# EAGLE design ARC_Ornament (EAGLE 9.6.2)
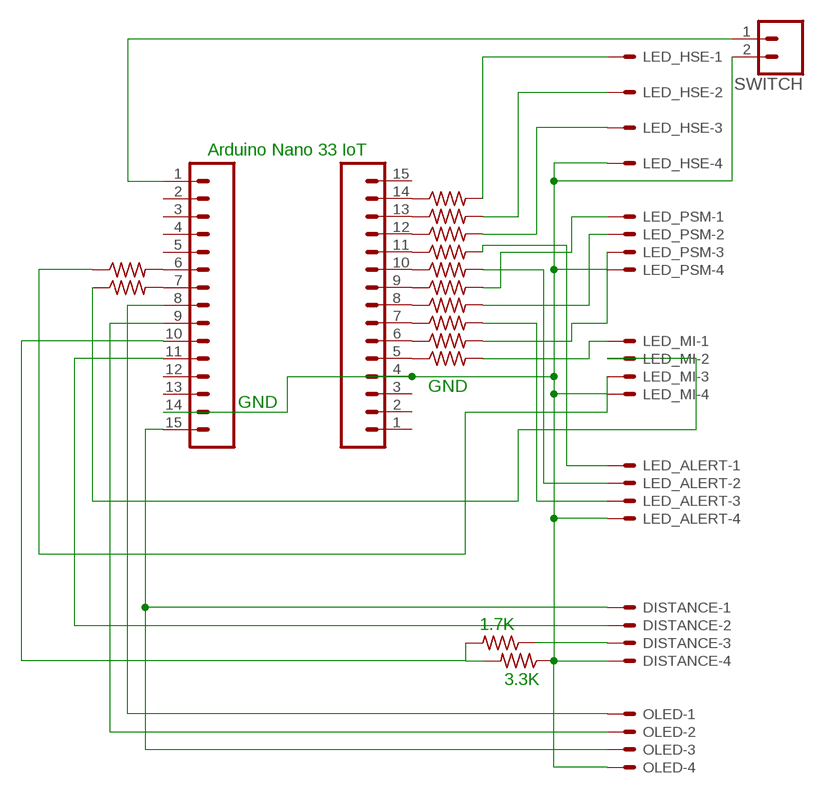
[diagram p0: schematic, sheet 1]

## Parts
1K7  R-US_0204/7  [0204/7]
3K3  R-US_0204/7  [0204/7]
DISTANCE  22-27-2041-04  [6410-04]
J1  CONN_15  [1X15]
J5  CONN_15  [1X15]
LED_ALERT  22-27-2041-04  [6410-04]
LED_HSE  22-27-2041-04  [6410-04]
LED_MI  22-27-2041-04  [6410-04]
LED_PSM  22-27-2041-04  [6410-04]
OLED  22-27-2041-04  [6410-04]
R1  R-US_0204/7  [0204/7]
R2  R-US_0204/7  [0204/7]
R3  R-US_0204/7  [0204/7]
R4  R-US_0204/7  [0204/7]
R5  R-US_0204/7  [0204/7]
R6  R-US_0204/7  [0204/7]
R7  R-US_0204/7  [0204/7]
R8  R-US_0204/7  [0204/7]
R9  R-US_0204/7  [0204/7]
R10  R-US_0204/7  [0204/7]
R11  R-US_0204/7  [0204/7]
R12  R-US_0204/7  [0204/7]
SWITCH  CONN_02  [1X02]

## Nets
GND: 3K3.1 DISTANCE.4 J1.4 J5.14 LED_ALERT.4 LED_HSE.4 LED_MI.4 LED_PSM.4 OLED.4 SWITCH.2
N$1: J1.5 R1.1
N$3: LED_HSE.1 R7.2
N$6: J1.6 R2.1
N$7: J1.8 R3.1
N$8: J1.9 R4.1
N$9: J1.12 R5.1
N$10: J1.13 R6.1
N$11: J1.14 R7.1
N$12: LED_PSM.2 R3.2
N$13: J5.6 R9.2
N$14: J5.7 R10.2
N$15: LED_PSM.3 R2.2
N$16: LED_MI.1 R1.2
N$17: LED_MI.2 R10.1
N$18: LED_PSM.1 R4.2
N$19: LED_MI.3 R9.1
N$20: J1.11 R8.1
N$21: J1.10 R11.1
N$22: J1.7 R12.1
N$23: LED_ALERT.3 R12.2
N$24: LED_ALERT.2 R11.2
N$25: LED_ALERT.1 R8.2
N$26: J5.9 OLED.2
N$27: DISTANCE.1 J5.15 OLED.3
N$28: J5.8 OLED.1
N$29: J5.1 SWITCH.1
N$30: DISTANCE.2 J5.11
N$31: 1K7.2 3K3.2 J5.10
N$32: 1K7.1 DISTANCE.3
N$33: LED_HSE.2 R6.2
N$34: LED_HSE.3 R5.2
Unconnected: J1.1 J1.2 J1.3 J1.15 J5.2 J5.3 J5.4 J5.5 J5.12 J5.13

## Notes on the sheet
- Arduino Nano 33 IoT
- GND
- GND
- 1.7K
- 3.3K

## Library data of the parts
1K7 3K3 R1-R12 = rcl:R-US_: RESISTOR, American symbol; SPICEPREFIX: R
DISTANCE LED_ALERT LED_HSE LED_MI LED_PSM OLED = sean-4pin-molexbr:22-?-04: CONNECTOR wire to board 2.54 mm (.1 inch) pitch header; MF: MOLEX; OC_FARNELL: unknown; OC_NEWARK: unknown
J1 J5 = SparkFun-Connectors:CONN_15: Multi connection point. Often used as Generic Header-pin footprint for 0.1 inch spaced/style header connections On any of the 0.1 inch spaced packages, you can populate with these: Break Away Headers - Straight (PRT-00116) Break Away Male Headers - Right Angle (PRT-00553) Female Headers (PRT-00115)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
SWITCH = SparkFun-Connectors:CONN_02: Multi connection point. Often used as Generic Header-pin footprint for 0.1 inch spaced/style header connections

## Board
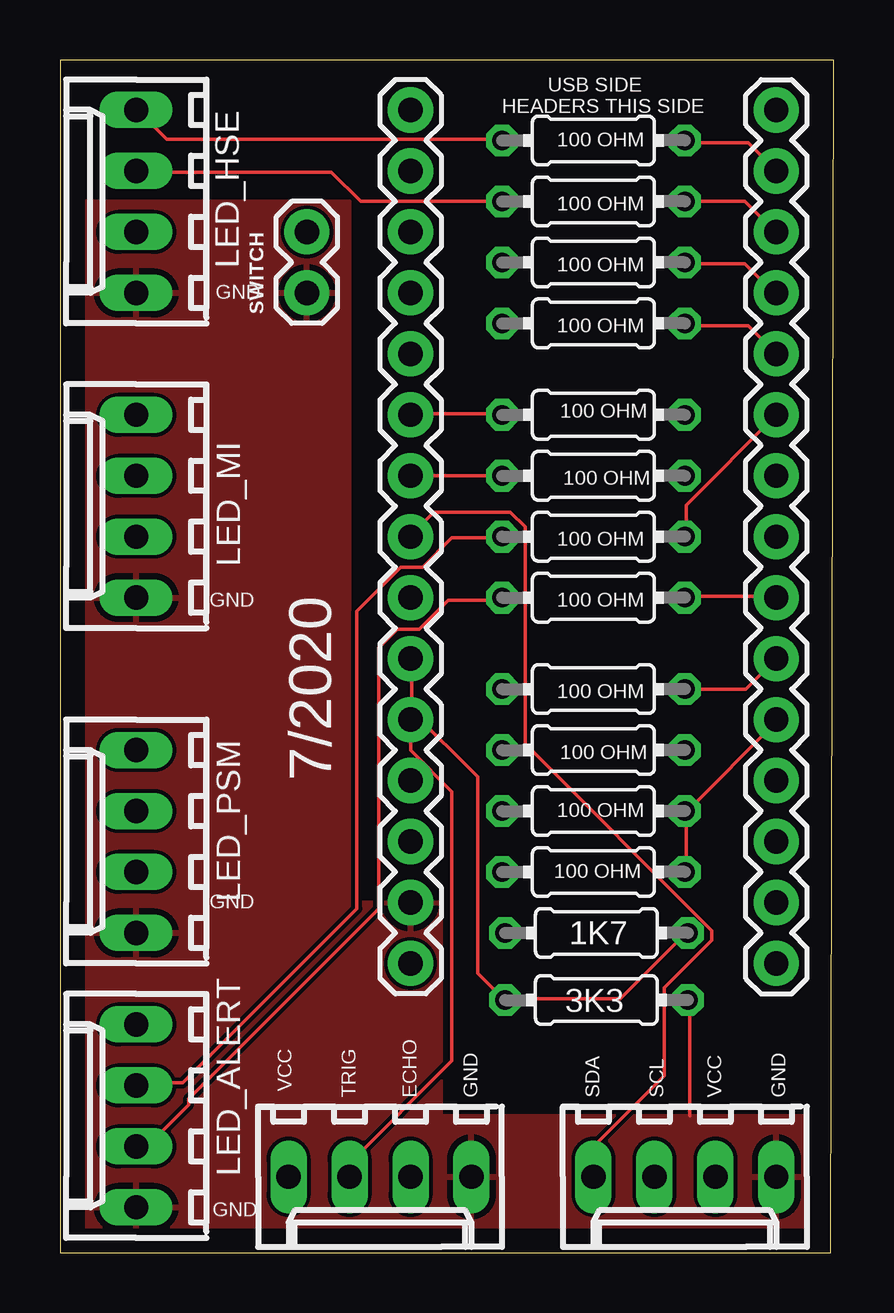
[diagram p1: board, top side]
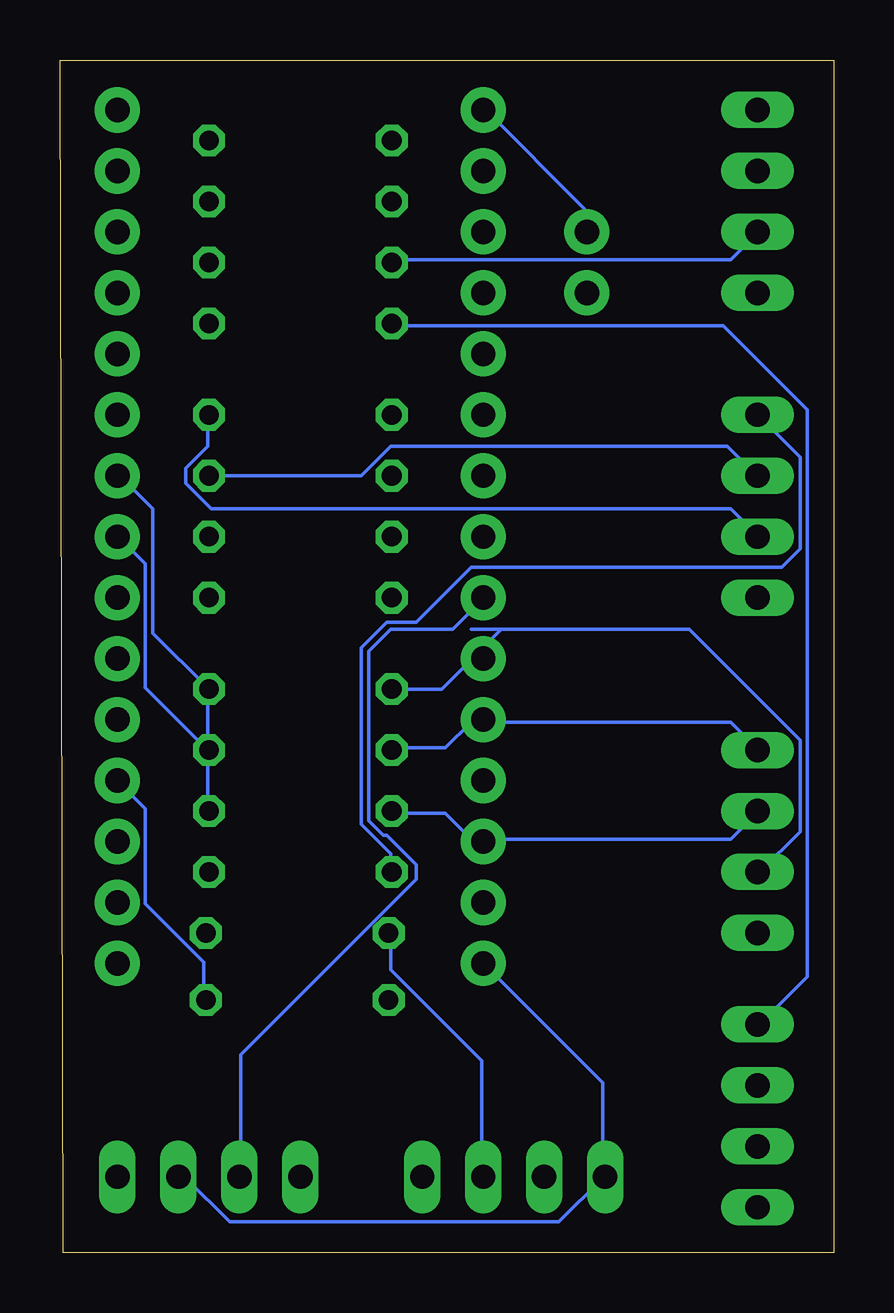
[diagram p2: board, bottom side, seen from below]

Size 32.24 x 49.71 mm. Coordinates in mm from the lower left corner, seen from the top.
Outline: 0,0 32.11,0 32.24,49.71 0,49.71 0,0
Copper layers (1*16): Top 0.035mm / dielectric 1.5mm / Bottom 0.035mm
Design rules "default": minimum track width 6mil, minimum drill 0.35mm, track to track 6mil, track to pad 6mil, pad to pad 6mil, via to via 6mil, smd to smd 6mil, copper to edge 40mil, drill to drill 6mil, minimum pad ring 10mil, minimum via ring 8mil, stop-mask expansion 4mil, vias tented up to drill 0mil, thermal gap 10mil

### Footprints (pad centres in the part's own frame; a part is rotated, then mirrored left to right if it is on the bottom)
0204/7 = drill 0.813 octagon: 1 -3.81,0; 2 3.81,0
6410-04 = drill 1.016 long: 1 3.81,0; 2 1.27,0; 3 -1.27,0; 4 -3.81,0
1X15 = drill 1.016 pad 1.88: 1 0,0; 2 2.54,0; 3 5.08,0; 4 7.62,0; 5 10.16,0; 6 12.7,0; 7 15.24,0; 8 17.78,0; 9 20.32,0; 10 22.86,0; 11 25.4,0; 12 27.94,0; 13 30.48,0; 14 33.02,0; 15 35.56,0
1X02 = drill 1.016 pad 1.88: 1 0,0; 2 2.54,0

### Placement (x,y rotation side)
1K7  22.35,13.34 0 top
3K3  22.35,10.54 180 top
DISTANCE  13.34,3.17 180 top
J1  29.84,12.06 90 top
J5  14.61,47.62 270 top
LED_ALERT  3.17,5.71 90 top
LED_HSE  3.17,43.81 90 top
LED_MI  3.17,31.12 90 top
LED_PSM  3.17,17.14 90 top
OLED  26.04,3.17 180 top
R1  22.23,15.88 180 top
R2  22.23,23.49 180 top
R3  22.23,18.41 180 top
R4  22.23,20.95 180 top
R5  22.23,41.27 180 top
R6  22.23,43.81 180 top
R7  22.23,46.35 180 top
R8  22.23,38.73 180 top
R9  22.23,34.93 180 top
R10  22.23,32.38 180 top
R11  22.23,29.84 180 top
R12  22.23,27.3 180 top
SWITCH  10.29,42.54 270 top

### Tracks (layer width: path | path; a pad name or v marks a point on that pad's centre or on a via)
GND
  Top 0.152: 26.24,5.71 26.24,10.44 3K3.1
  Bottom 0.152: J1.4 28.68,18.52 28.68,14.55 26.24,12.12 26.24,10.59 3K3.1
  pour Top: 0.63,0.63 31.12,0.63 31.12,5.71 15.88,5.71 15.88,14.6 12.07,14.6 12.07,43.81 0.63,43.81
N$1
  Top 0.152: R1.1 26.09,15.88 26.09,18.36 29.9,22.17 J1.5
N$3
  Top 0.152: R7.2 18.31,46.41 4.44,46.41 3.23,47.62 LED_HSE.1
N$6
  Top 0.152: J1.6 28.58,23.49 R2.1
N$7
  Bottom 0.152: R3.1 26.09,18.47 26.09,20.95 28.68,23.55 28.68,28.73 29.74,29.79 J1.8
N$8
  Bottom 0.152: R4.1 26.09,21.06 26.09,23.55 28.37,25.83 28.37,31.01 29.74,32.38 J1.9
N$9
  Top 0.152: R5.1 26.09,41.22 28.52,41.22 29.74,40.01 J1.12
N$10
  Top 0.152: R6.1 28.52,43.81 29.74,42.6 J1.13
N$11
  Top 0.152: J1.14 28.68,46.25 26.09,46.25 R7.1
N$12
  Bottom 0.152: R3.2 18.31,18.31 16.18,18.31 15.11,17.25 4.29,17.25 3.23,18.31 LED_PSM.2
N$13
  Top 0.152: R9.2 18.31,34.98 14.66,34.98 J5.6
N$14
  Top 0.152: J5.7 R10.2
N$15
  Bottom 0.152: R2.2 16.33,23.49 13.84,25.98 | 15.11,25.98 6.02,25.98 1.4,21.36 1.4,17.55 3.07,15.88 LED_PSM.3
N$16
  Bottom 0.152: LED_MI.1 1.4,33.15 1.4,29.34 2.16,28.57 15.11,28.57 17.4,26.29 18.62,26.29 19.69,25.22 19.69,17.86 18.47,16.64 18.47,15.88 R1.2
N$17
  Bottom 0.152: R10.1 19.69,32.38 18.47,33.6 4.44,33.6 3.23,32.38 LED_MI.2
N$18
  Bottom 0.152: R4.2 18.31,21.06 16.18,21.06 15.11,22.12 4.29,22.12 3.23,21.06 LED_PSM.1
N$19
  Bottom 0.152: R9.1 26.09,34.82 26.09,33.6 27,32.69 27,32.08 25.93,31.01 4.29,31.01 3.23,29.95 LED_MI.3
N$20
  Top 0.152: J1.11 28.68,38.63 26.09,38.63 R8.1
N$21
  Top 0.152: J1.10 26.09,31.17 26.09,29.95 R11.1
N$22
  Top 0.152: R12.1 26.09,27.36 29.74,27.36 J1.7
N$23
  Top 0.152: R12.2 18.31,27.2 16.18,27.2 14.96,25.98 14.05,25.98 13.28,25.22 13.28,14.35 5.36,6.43 5.36,6.17 3.68,4.5 3.23,4.5 LED_ALERT.3
N$24
  Top 0.152: R11.2 18.31,29.79 16.33,29.79 15.11,28.57 14.2,28.57 12.37,26.75 12.37,14.35 5.1,7.09 3.23,7.09 LED_ALERT.2
N$25
  Bottom 0.152: R8.2 18.31,38.63 4.6,38.63 1.09,35.13 1.09,11.51 3.07,9.52 LED_ALERT.1
N$26
  Bottom 0.152: OLED.2 24.71,3.28 24.71,8.25 17.4,15.57 17.4,16.18 18.62,17.4 18.77,17.4 19.38,18.01 19.38,25.07 18.47,25.98 15.88,25.98 14.66,27.2 J5.9
N$27
  Bottom 0.152: J5.15 9.63,7.09 9.63,3.28 DISTANCE.1 9.63,3.12 11.46,1.29 25.17,1.29 27,3.12 27.3,3.12 OLED.3
N$28
  Top 0.152: OLED.1 22.28,3.28 22.28,4.5 25.17,7.39 25.17,11.05 27.15,13.03 27.15,13.44 19.38,21.21 19.38,30.25 18.77,30.86 15.57,30.86 14.66,29.95 J5.8
N$29
  Bottom 0.152: SWITCH.1 10.39,42.6 10.39,43.51 14.5,47.62 J5.1
N$30
  Top 0.152: DISTANCE.2 12.07,3.73 16.33,8 16.33,19.23 14.61,20.95 J5.11
N$31
  Top 0.152: 1K7.2 26.09,13.34 23.34,10.59 18.62,10.59 3K3.2 18.47,10.59 17.4,11.66 17.4,19.84 14.66,22.58 14.66,24.71 J5.10
N$32
  Bottom 0.152: 1K7.1 18.47,13.34 18.47,11.81 14.66,8 14.66,3.28 DISTANCE.3
N$33
  Top 0.152: R6.2 12.52,43.81 11.3,45.03 3.23,45.03 LED_HSE.2
N$34
  Bottom 0.152: R5.2 18.31,41.38 4.29,41.38 3.23,42.44 LED_HSE.3

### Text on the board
tPlace: GND | GND | GND | VCC | TRIG | ECHO | GND | SDA | SCL | VCC | GND | GND
tNames: HEADERS THIS SIDE | USB SIDE | 100 OHM | 100 OHM | 100 OHM | 100 OHM | 100 OHM | 100 OHM | 100 OHM | 100 OHM | 100 OHM | 100 OHM | 7/2020 | 100 OHM | 100 OHM
silk_top: DISTANCE | OLED

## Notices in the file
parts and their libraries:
SparkFun-Connectors: Licensing: Creative Commons ShareAlike 4.0 International - https://creativecommons.org/licenses/by-sa/4.0
